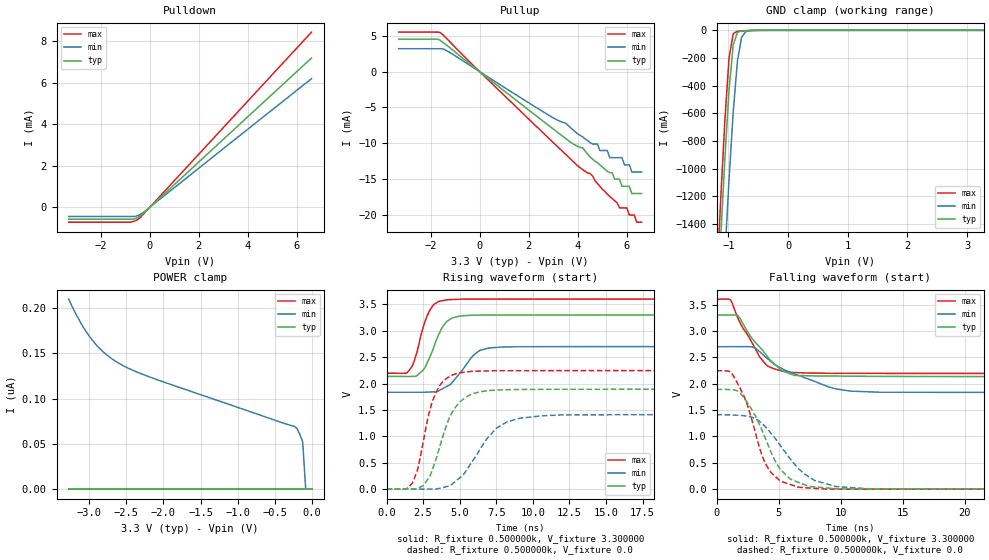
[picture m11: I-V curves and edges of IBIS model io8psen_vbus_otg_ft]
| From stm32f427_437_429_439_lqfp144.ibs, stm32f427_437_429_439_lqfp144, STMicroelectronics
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|   Model io8psen_vbus_otg_ft
[Model]  io8psen_vbus_otg_ft
Model_type 3-state
Polarity   Non-Inverting
Enable   Active-High
Vmeas =  1.650000V
Cref =   50.000000pF
Rref =   100.000000M
Vref =   0.0V
C_comp   3.300900pF   3.198000pF   3.426400pF
[Temperature Range]   25.000000   0.125000k   -40.000000
[Pullup Reference]   3.300000V   2.700000V   3.600000V
[Pulldown Reference]   0.0V   0.0V   0.0V
[POWER Clamp Reference]   3.300000V   2.700000V   3.600000V
[GND Clamp Reference]   0.0V   0.0V   0.0V
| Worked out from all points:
|   slope of the pulldown table from 0 to 0.495 V, typ, clamps not added: 915 ohm
|   slope of the pullup table from 0 to 0.495 V, typ, clamps not added: 371 ohm
|   GND clamp passes 1 mA (typ) near -0.61 V on its own axis
|   rising waveform, R_fixture 0.500000k, V_fixture 3.300000: 20-80 % time 1.08ns typ, 1.47ns min, 889ps max; typ from 2.13 V to 3.3 V
|   rising waveform, R_fixture 0.500000k, V_fixture 0.0: 20-80 % time 1.47ns typ, 2.14ns min, 1.15ns max; typ from 0 V to 1.89 V
|   falling waveform, R_fixture 0.500000k, V_fixture 3.300000: 20-80 % time 2.4ns typ, 4.43ns min, 1.99ns max; typ from 3.3 V to 2.13 V
|   falling waveform, R_fixture 0.500000k, V_fixture 0.0: 20-80 % time 2.3ns typ, 2.98ns min, 1.88ns max; typ from 1.89 V to 0 V
[Pulldown]
|Voltage   I(typ)   I(min)   I(max)
-3.3V     -568.8uA   -435.6uA   -711.6uA
-800mV    -568.8uA   -435.6uA   -711.6uA
-600mV    -538.7uA   -432.7uA   -651.9uA
-400mV    -425uA     -350.3uA   -505.8uA
6.6V      7.199mA    6.203mA    8.444mA
[Pullup]
|Voltage   I(typ)   I(min)   I(max)
-3.3V     4.529mA    3.197mA    5.513mA
-1.6V     4.34mA     3.197mA    5.455mA
3.5V      -9.319mA   -7.182mA   -11.52mA
4.8V      -12.7mA    -10.1mA    -15.6mA
4.9V      -13mA      -11mA      -16mA
5.2V      -13.9mA    -11mA      -17.1mA
5.3V      -14.1mA    -12mA      -17.4mA
5.8V      -16mA      -12mA      -19mA
6V        -16mA      -13mA      -19mA
6.1V      -16mA      -13mA      -20mA
6.2V      -17mA      -14mA      -20mA
6.6V      -17mA      -14mA      -21mA
[GND_clamp]
|Voltage   I(typ)   I(min)   I(max)
-3.3V     -9.429A    -9.432A    -9.904A
-1.2V     -2.113A    -2.844A    -1.842A
-1.13V    -1.502A    -2.228A    -1.224A
-1.06V    -927mA     -1.634A    -653.1mA
-990mV    -428.7mA   -1.078A    -200.2mA
-920mV    -105.4mA   -587.6mA   -23.28mA
-850mV    -14.68mA   -223.7mA   -6.667mA
-780mV    -4.207mA   -50.77mA   -4.248mA
-710mV    -2.321mA   -9.26mA    -2.639mA
-640mV    -1.305mA   -2.349mA   -1.385mA
3.28V     0A         0A         0A
[POWER_clamp]
|Voltage   I(typ)   I(min)   I(max)
-3.28V    0A         210.1nA    0A
-3.12V    0A         184.2nA    0A
-2.96V    0A         164.6nA    0A
-2.8V     0A         150.7nA    0A
-2.6V     0A         139nA      0A
-2.16V    0A         123.2nA    0A
-240mV    0A         69.7nA     0A
-200mV    0A         67.32nA    0A
-160mV    0A         60.72nA    0A
-120mV    0A         52.23nA    0A
-80mV     0A         0A         0A
0V        0A         0A         0A
[Ramp]
| variable   typ   min   max
dV/dt_r  1.13460/1.46339n   0.84588/2.14013n   1.34694/1.14432n
dV/dt_f  0.69930/2.39522n   0.51900/4.42742n   0.84306/1.98791n
R_load = 0.500000k
[Rising Waveform]
R_fixture= 0.500000k
V_fixture= 3.300000
V_fixture_min= 2.700000
V_fixture_max= 3.600000
|time   V(typ)   V(min)   V(max)
0s        2.135V     1.835V     2.195V
1.376ns   2.133V     1.835V     2.197V
2.127ns   2.159V     1.835V     2.637V
2.628ns   2.301V     1.835V     3.176V
3.003ns   2.528V     1.839V     3.406V
3.754ns   3.038V     1.89V      3.566V
4.254ns   3.2V       1.964V     3.589V
6.256ns   3.296V     2.603V     3.599V
7.758ns   3.299V     2.69V      3.599V
62.31ns   3.3V       2.7V       3.6V
[Rising Waveform]
R_fixture= 0.500000k
V_fixture= 0.0
V_fixture_min= 0.0
V_fixture_max= 0.0
|time   V(typ)   V(min)   V(max)
0s        15.8uV     12.44uV    8.086uV
1.752ns   -604.5uV   -56.76uV   105.5mV
2.503ns   62.2mV     -1.115mV   883.1mV
3.003ns   264.5mV    402.9uV    1.535V
3.504ns   674mV      6.377mV    1.895V
4.254ns   1.325V     57.38mV    2.125V
5.13ns    1.677V     241.4mV    2.208V
7.508ns   1.875V     1.153V     2.242V
10.64ns   1.889V     1.388V     2.244V
62.31ns   1.891V     1.41V      2.245V
[Falling Waveform]
R_fixture= 0.500000k
V_fixture= 3.300000
V_fixture_min= 2.700000
V_fixture_max= 3.600000
|time   V(typ)   V(min)   V(max)
0s        3.3V       2.7V       3.6V
1.126ns   3.303V     2.702V     3.588V
1.752ns   3.282V     2.702V     3.227V
3.003ns   2.817V     2.686V     2.715V
4.004ns   2.542V     2.494V     2.358V
5.255ns   2.249V     2.289V     2.241V
6.131ns   2.17V      2.199V     2.213V
9.635ns   2.144V     1.9V       2.196V
13.14ns   2.139V     1.838V     2.195V
62.31ns   2.135V     1.835V     2.195V
[Falling Waveform]
R_fixture= 0.500000k
V_fixture= 0.0
V_fixture_min= 0.0
V_fixture_max= 0.0
|time   V(typ)   V(min)   V(max)
0s        1.891V     1.41V      2.245V
1.502ns   1.877V     1.404V     2.089V
2.878ns   1.492V     1.362V     1.29V
3.629ns   1.137V     1.249V     664.4mV
4.379ns   706.6mV    1.06V      315.8mV
5.13ns    377.2mV    831mV      156mV
6.632ns   127mV      384.2mV    36.19mV
9.635ns   8.143mV    48.37mV    2.066mV
12.64ns   1.087mV    3.189mV    125.9uV
62.31ns   15.8uV     12.44uV    8.086uV
